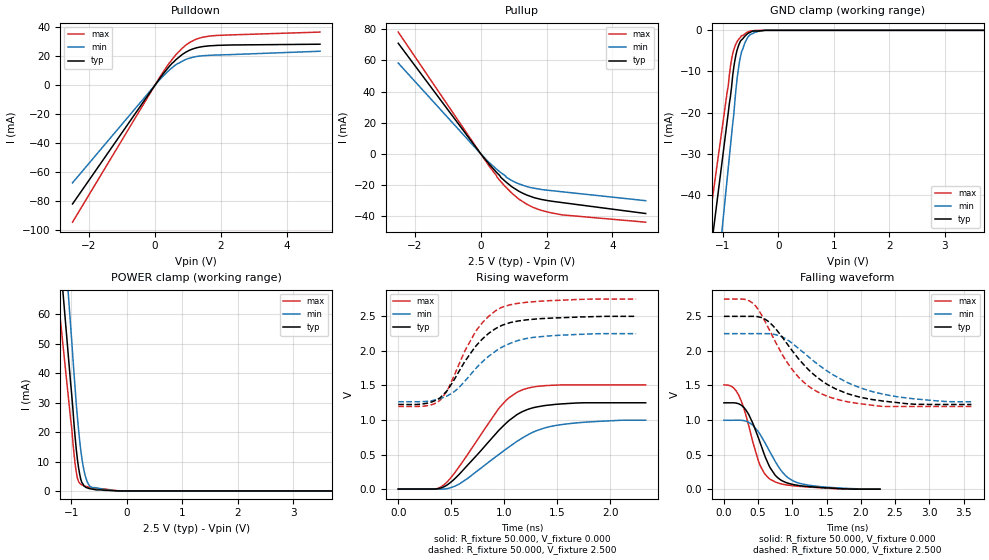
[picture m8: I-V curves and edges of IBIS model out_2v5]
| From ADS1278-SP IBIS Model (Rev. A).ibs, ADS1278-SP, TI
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[Model]   out_2v5
Model_type Output
Vref=0.000E+00
Rref=1.000E+06
Cref=2.000E-11
Vmeas=1.250E+00
C_comp   853.00E-15   853.00E-15   853.00E-15
[Voltage Range]   2.500E+00   2.250E+00   2.750E+00
[POWER Clamp Reference]   2.500E+00   2.250E+00   2.750E+00
[GND Clamp Reference]   0.000E+00   0.000E+00   0.000E+00
[Pullup Reference]   2.500E+00   2.250E+00   2.750E+00
[Pulldown Reference]   0.000E+00   0.000E+00   0.000E+00
[Temperature Range]   25   105   -40
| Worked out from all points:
|   slope of the pulldown table from 0 to 0.375 V, typ, clamps not added: 33.1 ohm
|   slope of the pullup table from 0 to 0.375 V, typ, clamps not added: 39.7 ohm
|   GND clamp passes 1 mA (typ) near -0.57 V on its own axis
|   POWER clamp passes 1 mA (typ) near -0.71 V on its own axis
|   rising waveform, R_fixture 50.000, V_fixture 0.000: 20-80 % time 455ps typ, 545ps min, 408ps max; typ from 0 V to 1.25 V
|   falling waveform, R_fixture 50.000, V_fixture 0.000: 20-80 % time 315ps typ, 373ps min, 272ps max; typ from 1.25 V to 0 V
|   rising waveform, R_fixture 50.000, V_fixture 2.500: 20-80 % time 362ps typ, 411ps min, 325ps max; typ from 1.23 V to 2.5 V
|   falling waveform, R_fixture 50.000, V_fixture 2.500: 20-80 % time 759ps typ, 940ps min, 621ps max; typ from 2.5 V to 1.23 V
[GND Clamp]
-2.5V     -191.9mA   -249.2mA   -169.5mA
-2.46V    -187.2mA   -243.8mA   -165.6mA
-920mV    -22.19mA   -36.21mA   -15.07mA
-860mV    -16.05mA   -28.12mA   -8.8mA
-820mV    -11.04mA   -22.73mA   -5.711mA
-760mV    -5.867mA   -14.27mA   -3.246mA
-720mV    -3.935mA   -9.67mA    -2.317mA
-660mV    -2.32mA    -5.225mA   -1.282mA
-560mV    -892.9uA   -1.947mA   -468.4uA
-420mV    -173uA     -504.4uA   -24.8uA
-220mV    0A         0A         0A
5V        0A         0A         0A
[Power Clamp]
-2.51V    371.9mA    448.5mA    299.1mA
-2.47V    362.2mA    438mA      291.8mA
-1.01V    36.39mA    55.69mA    24.1mA
-930mV    18.19mA    34.71mA    9.106mA
-890mV    10.82mA    25.18mA    4.361mA
-870mV    8.062mA    21.08mA    3.233mA
-810mV    2.897mA    11.18mA    2.06mA
-770mV    1.704mA    6.818mA    1.745mA
-730mV    1.176mA    4.026mA    1.5mA
-630mV    659.4uA    1.136mA    1.172mA
-190mV    38.95uA    0A         120.7uA
5.01V     0A         0A         0A
[Pullup]
-2.51V    70.94mA    58.24mA    78.11mA
70mV      -1.831mA   -1.599mA   -2.214mA
550mV     -13.37mA   -11.07mA   -16.35mA
610mV     -15.08mA   -12.06mA   -17.81mA
750mV     -17.76mA   -14.14mA   -21.13mA
790mV     -18.45mA   -15.21mA   -21.95mA
1.17V     -24.1mA    -19.32mA   -29.22mA
1.59V     -27.86mA   -21.92mA   -34.32mA
1.83V     -29.17mA   -22.77mA   -36.17mA
2.19V     -30.45mA   -23.66mA   -38.03mA
2.49V     -31.29mA   -24.34mA   -39.14mA
5.01V     -38.23mA   -30.01mA   -43.8mA
[Pulldown]
-2.5V     -81.84mA   -67.28mA   -94.4mA
200mV     6.379mA    5.141mA    7.464mA
460mV     13.6mA     10.86mA    15.89mA
620mV     17.19mA    13.82mA    20.63mA
940mV     22.78mA    17.77mA    27.65mA
1.28V     25.84mA    19.81mA    31.91mA
1.66V     27.09mA    20.57mA    33.79mA
5V        28.19mA    23.34mA    36.54mA
[Rising Waveform]
R_fixture = 50.000
V_fixture = 0.000
V_fixture_min = 0.000
V_fixture_max = 0.000
|  time   V(typ)   V(min)   V(max)
0s        0V         0V         0V
345ps     699.7uV    -200uV     699.1uV
435ps     35.92mV    1.5mV      66.03mV
590ps     237.9mV    87.07mV    355.9mV
955ps     859.1mV    507.8mV    1.178V
1.045ns   991.6mV    609.1mV    1.321V
1.145ns   1.099V     714.4mV    1.419V
1.31ns    1.189V     847.6mV    1.486V
1.505ns   1.228V     924.7mV    1.506V
2.335ns   1.249V     996.6mV    1.508V
[Falling Waveform]
R_fixture = 50.000
V_fixture = 0.000
V_fixture_min = 0.000
V_fixture_max = 0.000
|  time   V(typ)   V(min)   V(max)
0s        1.249V     996.6mV    1.508V
175ps     1.246V     997.7mV    1.427V
250ps     1.217V     996.6mV    1.283V
320ps     1.147V     984.7mV    1.073V
505ps     738.1mV    827mV      403.5mV
585ps     515.4mV    697.1mV    238.2mV
675ps     309.4mV    534.5mV    143.5mV
850ps     120.8mV    250.9mV    72.96mV
1.08ns    54.59mV    92.34mV    42.67mV
2.28ns    0V         0V         0V
[Rising Waveform]
R_fixture = 50.000
V_fixture = 2.500
V_fixture_min = 2.250
V_fixture_max = 2.750
|  time   V(typ)   V(min)   V(max)
0s        1.225V     1.264V     1.196V
280ps     1.245V     1.271V     1.208V
400ps     1.328V     1.311V     1.294V
455ps     1.413V     1.343V     1.407V
540ps     1.614V     1.424V     1.684V
730ps     2.065V     1.741V     2.279V
850ps     2.249V     1.917V     2.495V
970ps     2.363V     2.046V     2.625V
1.29ns    2.46V      2.198V     2.713V
2.245ns   2.5V       2.25V      2.75V
[Falling Waveform]
R_fixture = 50.000
V_fixture = 2.500
V_fixture_min = 2.250
V_fixture_max = 2.750
|  time   V(typ)   V(min)   V(max)
0s        2.5V       2.25V      2.75V
370ps     2.5V       2.25V      2.724V
470ps     2.499V     2.25V      2.64V
610ps     2.453V     2.25V      2.408V
1.015ns   1.98V      2.096V     1.708V
1.23ns    1.734V     1.92V      1.494V
1.455ns   1.549V     1.745V     1.366V
1.815ns   1.378V     1.537V     1.262V
2.295ns   1.279V     1.381V     1.199V
3.615ns   1.225V     1.264V     1.196V
[Ramp]
dV/dt_r   7.499E-01/4.538E-10   5.979E-01/5.452E-10   9.063E-01/4.067E-10
dV/dt_f   7.651E-01/7.578E-10   5.918E-01/9.393E-10   9.324E-01/6.201E-10
R_load = 50
